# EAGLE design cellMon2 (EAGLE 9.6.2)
DATABASE: Z:\Eigene Dateien\Anwendungsdaten\Eagle\partdb\exp.txt

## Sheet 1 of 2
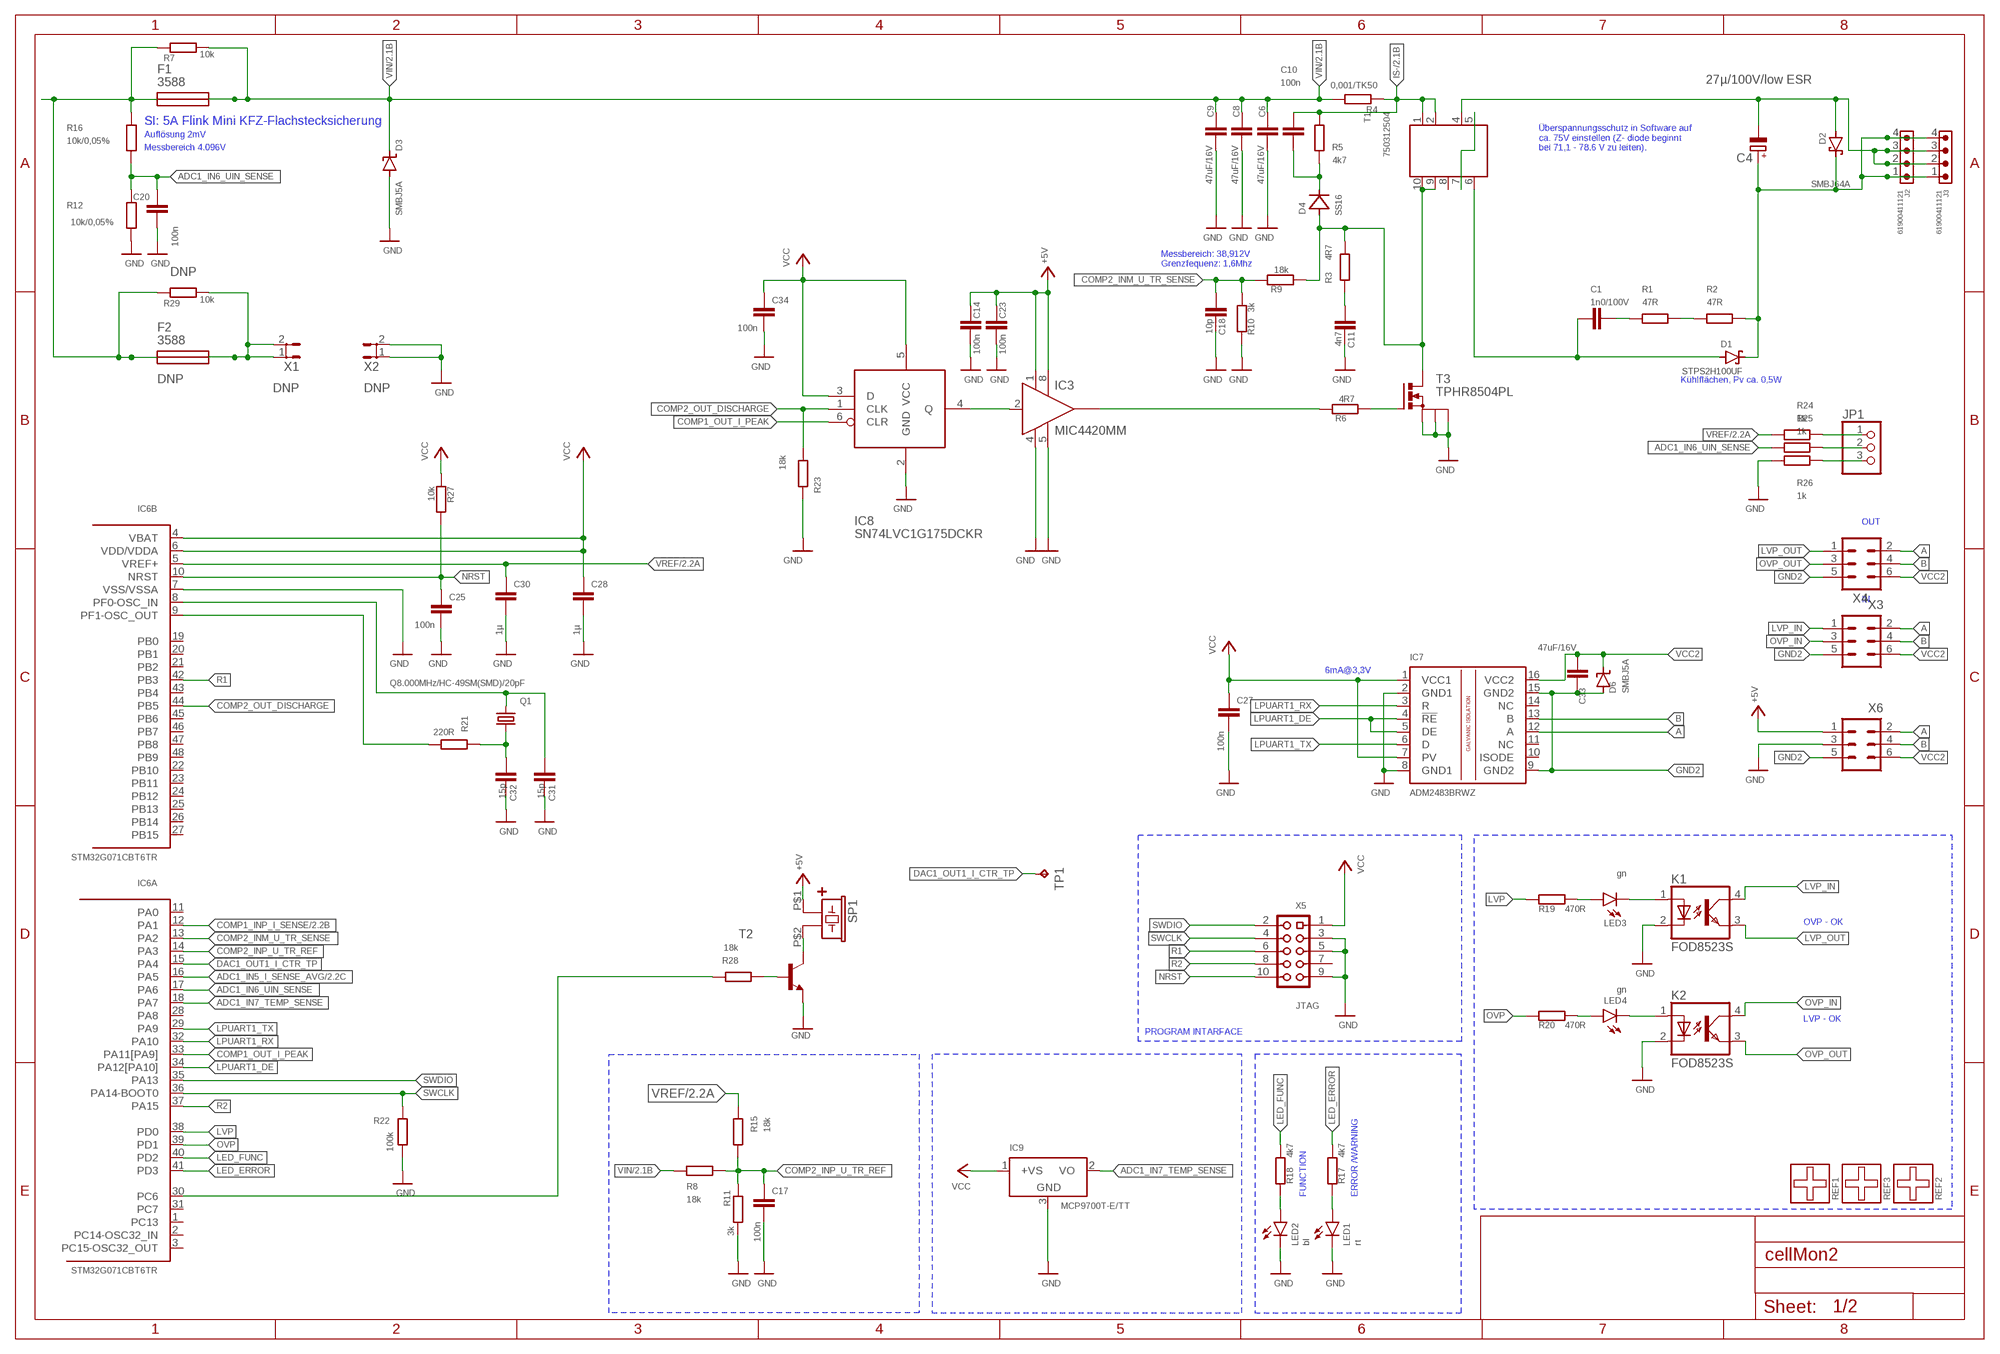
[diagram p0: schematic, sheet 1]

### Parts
C1  1n0/100V  C-EUC1206  [C1206]
C4  27µ/100V/low ESR  CPOL-EU153CLV-1010  [153CLV-1010]
C6  47uF/16V  C-EUC1210  [C1210]
C8  47uF/16V  C-EUC1210  [C1210]
C9  47uF/16V  C-EUC1210  [C1210]
C10  100n  C-EUC0603  [C0603]
C11  4n7  C-EUC0603K  [C0603K]
C14  100n  C-EUC0603K  [C0603K]
C17  100n  C-EUC0603K  [C0603K]
C18  10p  C-EUC0603  [C0603]
C20  100n  C-EUC0603K  [C0603K]
C23  100n  C-EUC0603K  [C0603K]
C25  100n  C-EUC0603K  [C0603K]
C27  100n  C-EUC0603K  [C0603K]
C28  1µ  C-EUC0603  [C0603]
C30  1µ  C-EUC0603  [C0603]
C31  15p  C-EUC0805  [C0805]
C32  15p  C-EUC0805  [C0805]
C33  47uF/16V  C-EUC1210  [C1210]
C34  100n  C-EUC0603K  [C0603K]
D1  STPS2H100UF  SCHOTTKY-DIODESMD  [SMB]
D2  SMBJ64A  SCHOTTKY-DIODESMD  [SMB]
D3  SMBJ5A  SUPPRESSOR-SMBJ  [SMBJ]
D4  SS16  MBRA340T3  [SMA]
D6  SMBJ5A  SUPPRESSOR-SMBJ  [SMBJ]
F1  3588  3588NORMAL  [3588]
F2  3588  3588NORMAL  [3588]
IC3  MIC4420MM  [MSOP8]
IC6  STM32G071CBT6TR  STM32G070CB  [LQFP48]
IC7  ADM2483BRWZ  ISO1176  [SO-16DW]
IC8  SN74LVC1G175DCKR  1G175  [SOT65P210X110-6N]
IC9  MCP9700T-E/TT  LM50  [SOT23]
J2  61900411121  61900411121  [61900411121]
J3  61900411121  61900411121  [61900411121]
JP1  PINHD-1X3  [1X03]
K1  FOD8523S  LTV816S  [SMD4]
K2  FOD8523S  LTV816S  [SMD4]
LED1  rt  LEDCHIPLED_0603  [CHIPLED_0603]
LED2  bl  LEDCHIPLED_0603  [CHIPLED_0603]
LED3  gn  LEDCHIPLED_0603  [CHIPLED_0603]
LED4  gn  LEDCHIPLED_0603  [CHIPLED_0603]
Q1  Q8.000MHz/HC-49SM(SMD)/20pF  CRYSTALHC49UP  [HC49UP]
R1  47R  R-EU_R1206  [R1206]
R2  47R  R-EU_R1206  [R1206]
R3  4R7  R-EU_R1206  [R1206]
R4  0,001/TK50  R-EU_R2512  [R2512]
R5  4k7  R-EU_R1206  [R1206]
R6  4R7  R-EU_R0603  [R0603]
R7  10k  R-EU_R0603  [R0603]
R8  18k  R-EU_R0603  [R0603]
R9  18k  R-EU_R0603  [R0603]
R10  3k  R-EU_R0603  [R0603]
R11  3k  R-EU_R0603  [R0603]
R12  10k/0,05%  R-EU_R0603  [R0603]
R15  18k  R-EU_R0603  [R0603]
R16  10k/0,05%  R-EU_R0603  [R0603]
R17  4k7  R-EU_R0603  [R0603]
R18  4k7  R-EU_R0603  [R0603]
R19  470R  R-EU_R0603  [R0603]
R20  470R  R-EU_R0603  [R0603]
R21  220R  R-EU_R0603  [R0603]
R22  100k  R-EU_R0603  [R0603]
R23  18k  R-EU_R0603  [R0603]
R24  1k  R-EU_R0603  [R0603]
R25  1k  R-EU_R0603  [R0603]
R26  1k  R-EU_R0603  [R0603]
R27  10k  R-EU_R0603  [R0603]
R28  18k  R-EU_R0603  [R0603]
R29  10k  R-EU_R0603  [R0603]
REF1  FIDUCIAL70UM_VERSION  [REF-DRUCK_FOR70UMCU]
REF2  FIDUCIAL70UM_VERSION  [REF-DRUCK_FOR70UMCU]
REF3  FIDUCIAL70UM_VERSION  [REF-DRUCK_FOR70UMCU]
SP1  LOUDITY_SPB45  [SPB45]
T1  750312504  WE-DSL_750050702  [WE_EP13_SMD_9PIN]
T2  MMBT2222ALT1-NPN-SOT23-BEC  [SOT23-BEC]
T3  TPHR8504PL  [DSOP8]
TP1  TPTP10R  [TP10R]
X1  ST6,3  [ST6,3]
X2  ST6,3  [ST6,3]
X3  ML6  [ML6]
X4  ML6  [ML6]
X5  JTAG  PF2X5SMD1.27MM  [PF2X5SMD50MIL]
X6  ML6  [ML6]

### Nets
+: C1.1 D1.A T1.6
+5V: C14.1 C23.1 IC3.1(VS) IC3.8(VS1) SP1.P$1(1P) X6.1 ; also sheet 2
+UB: F1.1A F1.1B F2.1A F2.1B R7.1 R16.1 R29.1
A: IC7.12(A) X3.2 X4.2 X6.2
ADC1_IN5_I_SENSE_AVG: IC6.16(A:PA5) ; also sheet 2
ADC1_IN6_UIN_SENSE: C20.1 IC6.17(A:PA6) R12.1 R16.2 R25.1
ADC1_IN6_UIN_SENSE_: JP1.2 R25.2
ADC1_IN7_TEMP_SENSE: IC6.18(A:PA7) IC9.2(VO)
B: IC7.13(B) X3.4 X4.4 X6.4
COMP1_INP_I_SENSE: IC6.12(A:PA1) ; also sheet 2
COMP1_OUT_I_PEAK: IC6.33(A:PA11[PA9]) IC8.6(CLR)
COMP2_INM_U_TR_SENSE: C18.1 IC6.13(A:PA2) R9.1 R10.2
COMP2_INP_U_TR_REF: C17.1 IC6.14(A:PA3) R8.2 R11.1 R15.2
COMP2_OUT_DISCHARGE: IC6.44(B:PB5) IC8.1(CLK) R23.2
DAC1_OUT1_I_CTR_TP: IC6.15(A:PA4) TP1.TP
GND: C6.2 C8.2 C9.2 C11.2 C14.2 C17.2 C18.2 C20.2 C23.2 C25.2 C27.2 C28.2 C30.2 C31.1 C32.1 C34.2 D3.A IC3.4(GND) IC3.5(GND1) IC6.7(B:VSS/VSSA) IC7.2(GND1) IC7.8(GND1) IC8.2(GND) IC9.3(GND) K1.2(C) K2.2(C) LED1.C LED2.C R10.1 R11.2 R12.2 R22.2 R23.1 R26.1 T2.E T3.S@1(S) T3.S@2(S) T3.S@3(S) X2.1 X2.2 X5.3 X5.5 X5.9 X6.3 ; also sheet 2
GND2: C33.1 D6.A IC7.9(GND2) IC7.15(GND2) X3.5 X4.5 X6.5
IS-: C10.1 R4.1 R5.2 T1.1 T1.2 ; also sheet 2
LED_ERROR: IC6.41(A:PD3) R17.1
LED_FUNC: IC6.40(A:PD2) R18.1
LPUART1_DE: IC6.34(A:PA12[PA10]) IC7.4(!RE) IC7.5(DE)
LPUART1_RX: IC6.32(A:PA10) IC7.3(R)
LPUART1_TX: IC6.29(A:PA9) IC7.6(D)
LVP: IC6.38(A:PD0) R19.1
LVP_IN: K1.4(COL) X3.1
LVP_OUT: K1.3(EMIT) X4.1
N$1: IC3.6(OUT) R6.1
N$2: R1.2 R2.1
N$3: C31.2 IC6.8(B:PF0-OSC_IN) Q1.2
N$5: C1.2 R1.1
N$7: C4.- D2.A J2.2 J2.3 J3.2 J3.3 T1.4
N$8: IC3.2(IN) IC8.4(Q)
N$9: IC6.9(B:PF1-OSC_OUT) R21.2
N$10: SP1.P$2(2N) T2.C
N$11: T1.5 T1.7
N$12: C32.2 Q1.1 R21.1
N$16: R28.2 T2.B
N$17: C4.+ D1.C D2.C J2.1 J2.4 J3.1 J3.4 R2.2
N$18: LED4.A R20.2
N$19: LED3.A R19.2
N$20: R6.2 T3.G
N$21: JP1.3 R26.2
N$23: C11.1 R3.1
N$24: D4.A R3.2 R9.2 T1.9 T1.10 T3.D
N$25: C10.2 D4.C R5.1
N$26: IC6.30(A:PC6) R28.1
N$28: F2.2A F2.2B R29.2 X1.1 X1.2
N$31: LED2.A R18.2
N$34: LED1.A R17.2
N$35: K2.1(A) LED4.C
N$36: K1.1(A) LED3.C
NRST: C25.1 IC6.10(B:NRST) R27.1 X5.10
OVP: IC6.39(A:PD1) R20.1
OVP_IN: K2.4(COL) X3.3
OVP_OUT: K2.3(EMIT) X4.3
R1: IC6.42(B:PB3) X5.6
R2: IC6.37(A:PA15) X5.8
SWCLK: IC6.36(A:PA14-BOOT0) R22.1 X5.4
SWDIO: IC6.35(A:PA13) X5.2
VCC: C27.1 C28.1 C34.1 IC6.4(B:VBAT) IC6.6(B:VDD/VDDA) IC7.1(VCC1) IC7.7(PV) IC8.3(D) IC8.5(VCC) IC9.1(+VS) R27.2 X5.1 ; also sheet 2
VCC2: C33.2 D6.C IC7.16(VCC2) X3.6 X4.6 X6.6
VIN: C6.1 C8.1 C9.1 D3.C F1.2A F1.2B R4.2 R7.2 R8.1 ; also sheet 2
VREF: C30.1 IC6.5(B:VREF+) R15.1 R24.1 ; also sheet 2
VREF_: JP1.1 R24.2
Unconnected: IC3.7(OUT) IC6.1(A:PC13) IC6.2(A:PC14-OSC32_IN) IC6.3(A:PC15-OSC32_OUT) IC6.11(A:PA0) IC6.19(B:PB0) IC6.20(B:PB1) IC6.21(B:PB2) IC6.22(B:PB10) IC6.23(B:PB11) IC6.24(B:PB12) IC6.25(B:PB13) IC6.26(B:PB14) IC6.27(B:PB15) IC6.28(A:PA8) IC6.31(A:PC7) IC6.43(B:PB4) IC6.45(B:PB6) IC6.46(B:PB7) IC6.47(B:PB8) IC6.48(B:PB9) IC7.10(ISODE) IC7.11(NC) IC7.14(NC) REF1.P$1 REF2.P$1 REF3.P$1 T1.8 X5.7

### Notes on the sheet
- SI: 5A Flink Mini KFZ-Flachstecksicherung
- Auflösung 2mV
- Messbereich 4.096V
- Überspannungsschutz in Software auf
  ca. 75V einstellen (Z- diode beginnt 
  bei 71,1 - 78.6 V zu leiten).
- Messbereich: 38,912V
- Grenzfequenz: 1,6Mhz
- Kühlflächen, Pv ca. 0,5W
- OUT
- IN
- 6mA@3,3V
- OVP - OK
- LVP - OK
- PROGRAM INTARFACE
- FUNCTION | ERROR /WARNING

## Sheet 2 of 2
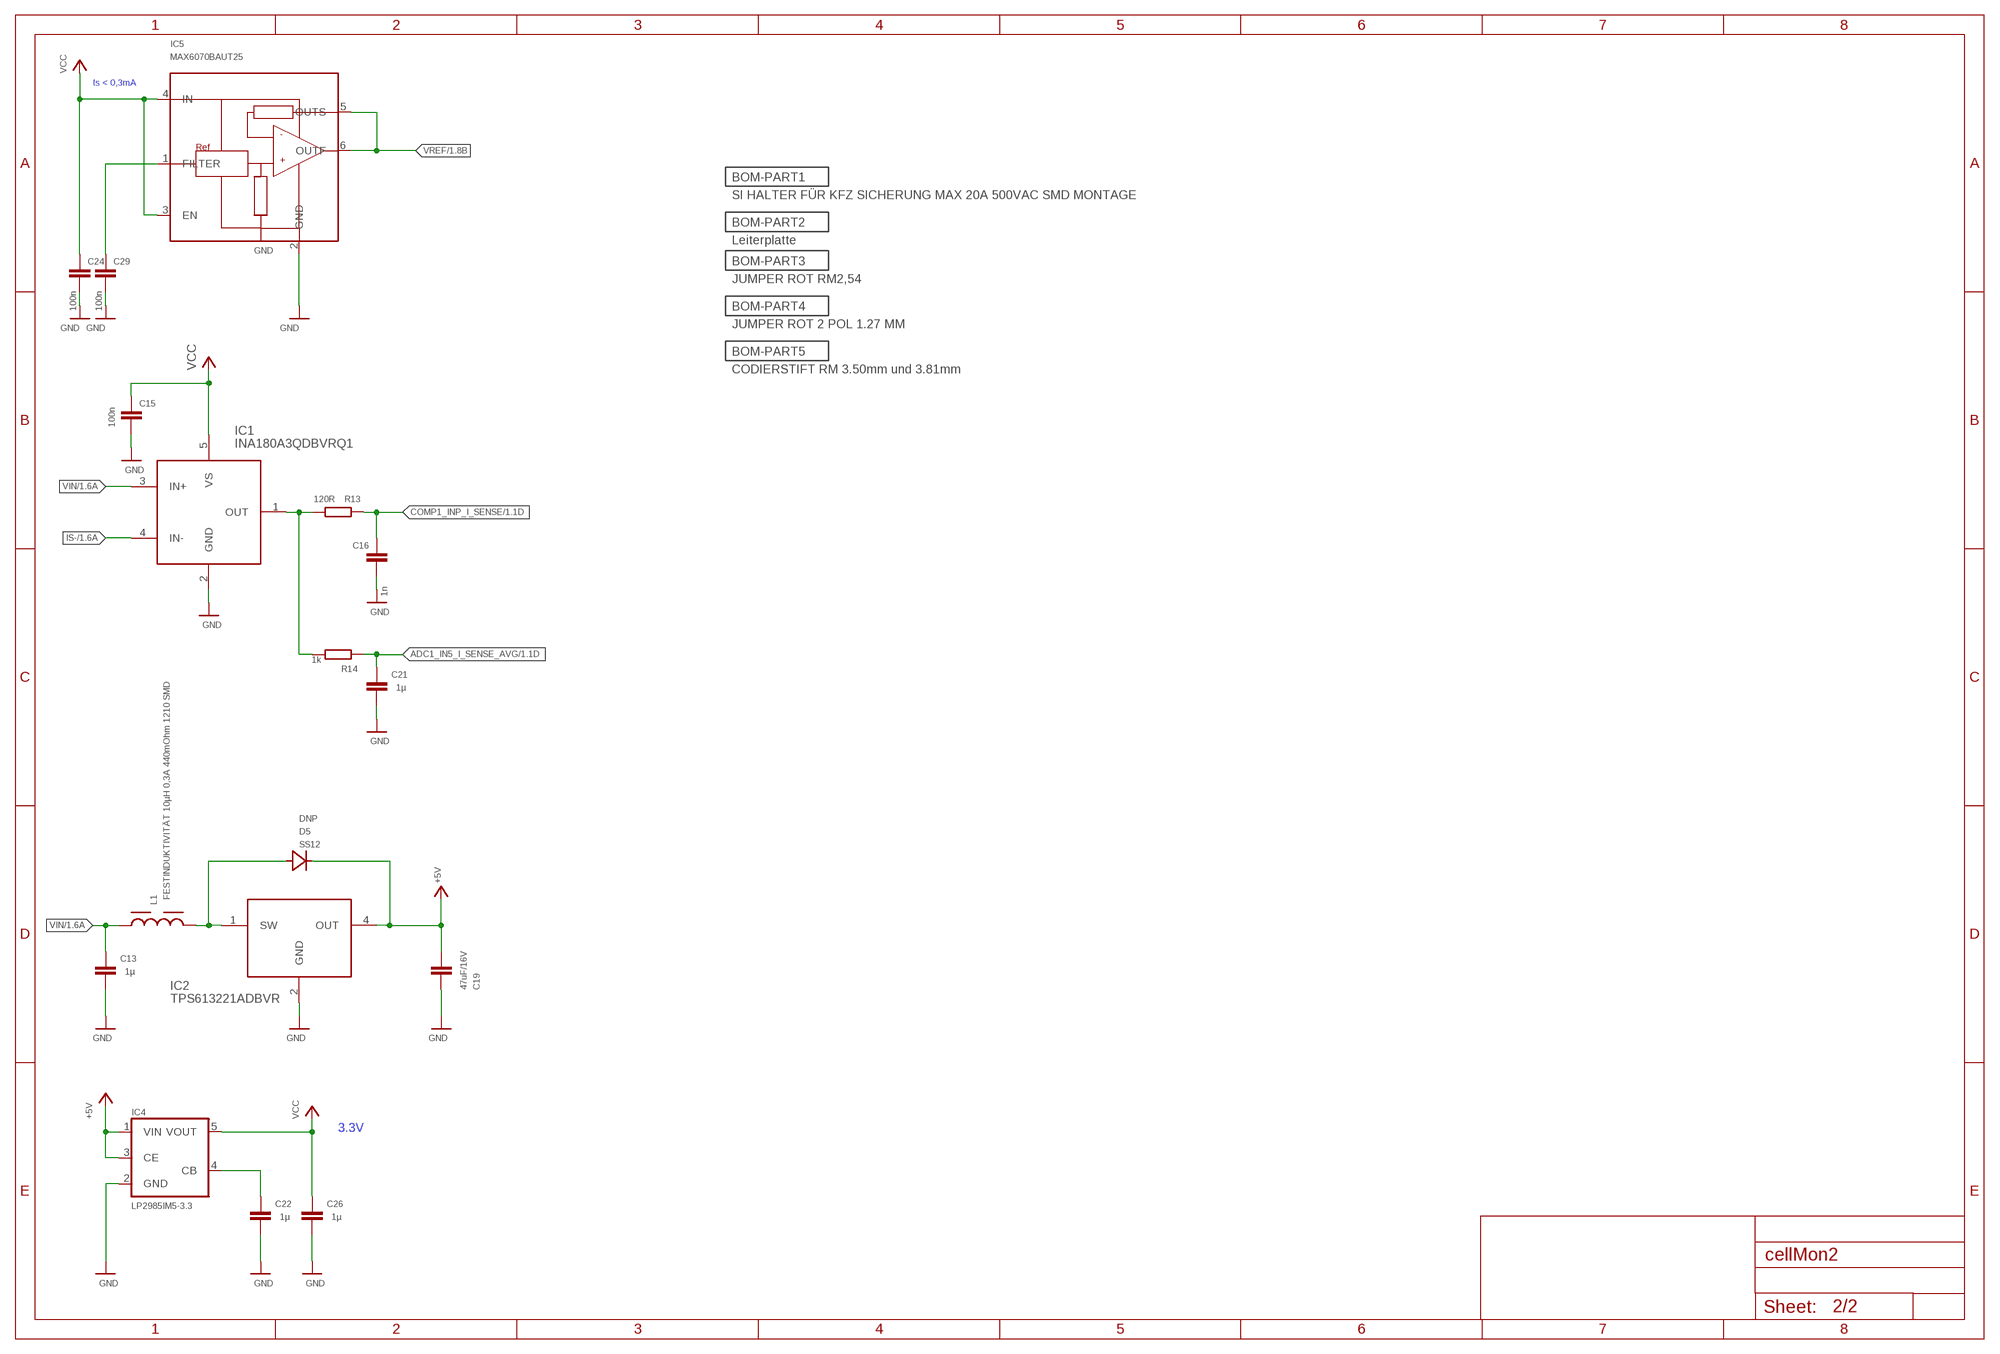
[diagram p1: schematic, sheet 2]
BOM-PART1 (BOM-PART): BOM: INCLUDE; PARTNO: EM008; QTY: 1
BOM-PART2 (BOM-PART): BOM: INCLUDE; PARTNO: PT057; QTY: 1
BOM-PART3 (BOM-PART): BOM: INCLUDE; PARTNO: CON085; QTY: 1
BOM-PART4 (BOM-PART): BOM: INCLUDE; PARTNO: CON363; QTY: 1
BOM-PART5 (BOM-PART): BOM: INCLUDE; PARTNO: CON441; QTY: 1

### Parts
C13  1µ  C-EUC0603  [C0603]
C15  100n  C-EUC0603K  [C0603K]
C16  1n  C-EUC0603  [C0603]
C19  47uF/16V  C-EUC1210  [C1210]
C21  1µ  C-EUC0603  [C0603]
C22  1µ  C-EUC0603  [C0603]
C24  100n  C-EUC0603K  [C0603K]
C26  1µ  C-EUC0603  [C0603]
C29  100n  C-EUC0603K  [C0603K]
D5  SS12  MBRA340T3  [SMA]
IC1  INA180A3QDBVRQ1  INA180A  [SOT95P280X110-5N]
IC2  TPS613221ADBVR  TPS613221ADBV  [SOT95P280X110-5N]
IC4  LP2985IM5-3.3  TS520529  [SOT25]
IC5  MAX6070BAUT25  MAX6070  [SOT23-6]
L1  FESTINDUKTIVITÄT 10µH 0,3A 440mOhm 1210 SMD  WE-LQS_3015_74404032022  [WE-LQS_3015]
R13  120R  R-EU_R0603  [R0603]
R14  1k  R-EU_R0603  [R0603]

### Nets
+5V: C19.1 D5.C IC2.4(OUT) IC4.1(VIN) IC4.3(CE) ; also sheet 1
ADC1_IN5_I_SENSE_AVG: C21.1 R14.1 ; also sheet 1
COMP1_INP_I_SENSE: C16.1 R13.1 ; also sheet 1
GND: C13.2 C15.2 C16.2 C19.2 C21.2 C22.2 C24.2 C26.2 C29.2 IC1.2(GND) IC2.2(GND) IC4.2(GND) IC5.2(GND) ; also sheet 1
IS-: IC1.4(IN-) ; also sheet 1
N$4: D5.A IC2.1(SW) L1.2
N$6: C22.1 IC4.4(CB)
N$14: IC1.1(OUT) R13.2 R14.2
N$22: C29.1 IC5.1(FILTER)
VCC: C15.1 C24.1 C26.1 IC1.5(VS) IC4.5(VOUT) IC5.3(EN) IC5.4(IN) ; also sheet 1
VIN: C13.1 IC1.3(IN+) L1.1 ; also sheet 1
VREF: IC5.5(OUTS) IC5.6(OUTF) ; also sheet 1

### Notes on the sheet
- Is < 0,3mA
- 3.3V

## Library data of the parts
C1 = rcl:C-EU: CAPACITOR, European symbol; PARTNO: C407; SPICEPREFIX: C
C4 = rcl:CPOL-EU: POLARIZED CAPACITOR, European symbol; PARTNO: C448; SPICEPREFIX: C
C6 C8 C9 C19 C33 = rcl:C-EU: CAPACITOR, European symbol; PARTNO: C219; SPICEPREFIX: C
C10 = rcl:C-EU: CAPACITOR, European symbol; PARTNO: C059; SPICEPREFIX: C
C11 = rcl:C-EU: CAPACITOR, European symbol; PARTNO: C051; SPICEPREFIX: C
C13 C21 C22 C26 C28 C30 = rcl:C-EU: CAPACITOR, European symbol; PARTNO: C079; SPICEPREFIX: C
C14 C15 C17 C20 C23-C25 C27 C29 C34 = rcl:C-EU: CAPACITOR, European symbol; PARTNO: C067; SPICEPREFIX: C
C16 = rcl:C-EU: CAPACITOR, European symbol; PARTNO: C043; SPICEPREFIX: C
C18 = rcl:C-EU: CAPACITOR, European symbol; PARTNO: C427; SPICEPREFIX: C
C31 C32 = resistor:C-EU: CAPACITOR, European symbol; PARTNO: C249
D1 = diode:SCHOTTKY-DIODE: Schottky Diode; PARTNO: D093
D2 = diode:SCHOTTKY-DIODE: Schottky Diode; PARTNO: D203
D3 D6 = diode:SUPPRESSOR-: Suppressor diode; PARTNO: D087
D4 = diode:MBRA340T3: Surface Mount Schottky Power Rectifier; PARTNO: D089
D5 = diode:MBRA340T3: Surface Mount Schottky Power Rectifier; DNP: T; PARTNO: D090
F1 = fuse_keystone_3568:3588; PARTNO: EM011
F2 = fuse_keystone_3568:3588; DNP: T; PARTNO: EM011
IC1 = ina180:INA180: Unidrectional current Sense Verstärkung 20/50/100/200; PARTNO: IC325
IC2 = TPS613221:TPS613221; PARTNO: IC328
IC3 = my_transistor-power:MIC4420: 6A-Peak Low-Side MOSFET Driver Bipolar/CMOS/DMOS Process http://www.micrel.com/_PDF/mic4420.pdf; PARTNO: IC039
IC4 = v-reg:TS5205: 150mA Low Noise LDO Voltage Regulator with Enable TSC [Taiwan Semiconductor Company, Ltd] Source: http://www.taiwansemi.com .. 5205_0409c.pdf; PARTNO: IC026
IC5 = max6070:MAX6070; PARTNO: IC326
IC6 = STM32G070CB:STM32G070CB: Arm® Cortex®-M0+ 32-bit MCU, 128 KB Flash, 36 KB RAM, 4x USART, timers, ADC, comm. I/Fs, 2.0-3.6V; PARTNO: IC321
IC7 = texas:ISO1176: ISOLATED RS-485 PROFIBUS TRANSCEIVER Source: Data sheet; MPN: ISO1176DW; OC_FARNELL: 1755037; OC_NEWARK: 13N4111; PARTNO: IC002
IC8 = 74LVC1G175:1G175: D Flip-Flop mit Reset im SC70 Gehäuse (6-pin); PARTNO: IC329
IC9 = linear:LM50: SOT-23 Single-Supply Centigrade Temperature Sensor Vout = (10mV/°C x Temp °C) +5mmmV Source: http://cache.national.com/ds/LM/LM50.pdf; PARTNO: IC040
J2 J3 = Wurth_Connectors_WR-WTB:61900411121: WR-WTB 2.54 mm Male Locking Header KIND PROPERTIES: Pitch:2.54 mm Gender:Male MATERIAL PROPERTIES: Insulator Material :PA66 Insulator Flammability Rating:UL94 V-0 Insulator Color:Beige Contact Material:Copper Alloy Contact Plating:Tin Contact Type:Stamped GENERAL INFORMATION Operating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; CONTACT-RESISTANCE: 20mOhm; DATASHEET-URL: https://www.we-online.com/redexpert/spec/61900411121?ae; GENDER: Male; L: 10.16mm; MOUNT: THT; PACKAGING: Bag; PART-NUMBER: 61900411121; PCB-CABLE-PANEL: PCB; PINS: 4; PITCH: 2.54mm; TYPE: Vertical; WORKING-VOLTAGE: 250V(AC)
JP1 = pinhead:PINHD-1X3: PIN HEADER; PARTNO: CON031
K1 K2 = optocoupler:LTV816: OPTO COUPLER Source: LITEON, LTV816.pdf; OC_FARNELL: unknown; OC_NEWARK: unknown; PARTNO: IC053
L1 = Wurth_Power Magnetics_WE-LQS:WE-LQS_3015: WE-LQS SMD Power Inductor; DATASHEET-URL: https://www.we-online.com/catalog/datasheet/74404032022.pdf; FRES: 75MHz; IR: 1.8A; ISAT: 1.7A; PART-NUMBER: 74404032022; PARTNO: L114; RDC: 50mOhm; VALUE: uH2.2
LED1 = led:LED: LED; PARTNO: D079
LED2 = led:LED: LED; PARTNO: D077
LED3 LED4 = led:LED: LED; PARTNO: D078
Q1 = crystal:CRYSTAL: CRYSTAL; OC_FARNELL: unknown; OC_NEWARK: unknown; PARTNO: Q003
R1 R2 = rcl:R-EU_: RESISTOR, European symbol; PARTNO: R574; SPICEPREFIX: R
R3 = rcl:R-EU_: RESISTOR, European symbol; PARTNO: R550; SPICEPREFIX: R
R4 = rcl:R-EU_: RESISTOR, European symbol; PARTNO: R826; SPICEPREFIX: R
R5 = rcl:R-EU_: RESISTOR, European symbol; PARTNO: R622; SPICEPREFIX: R
R6 = rcl:R-EU_: RESISTOR, European symbol; PARTNO: R141; SPICEPREFIX: R
R7 R27 = rcl:R-EU_: RESISTOR, European symbol; PARTNO: R221; SPICEPREFIX: R
R8 R9 R15 R23 R28 = rcl:R-EU_: RESISTOR, European symbol; PARTNO: R227; SPICEPREFIX: R
R10 R11 = rcl:R-EU_: RESISTOR, European symbol; PARTNO: R208; SPICEPREFIX: R
R12 R16 = rcl:R-EU_: RESISTOR, European symbol; PARTNO: R869; SPICEPREFIX: R
R13 = rcl:R-EU_: RESISTOR, European symbol; PARTNO: R175; SPICEPREFIX: R
R14 R24-R26 = rcl:R-EU_: RESISTOR, European symbol; PARTNO: R197; SPICEPREFIX: R
R17 R18 = rcl:R-EU_: RESISTOR, European symbol; PARTNO: R213; SPICEPREFIX: R
R19 R20 = rcl:R-EU_: RESISTOR, European symbol; PARTNO: R189; SPICEPREFIX: R
R21 = resistor:R-EU_: RESISTOR, European symbol; PARTNO: R181
R22 = resistor:R-EU_: RESISTOR, European symbol; PARTNO: R245
R29 = rcl:R-EU_: RESISTOR, European symbol; DNP: T; PARTNO: R221; SPICEPREFIX: R
REF1-REF3 = Fiducial (1):FIDUCIAL; BOM: EXCLUDE
SP1 = mBuzzer:LOUDITY_SPB45
T1 = Wuerth_Elektronik_eiSos_V6:WE-DSL_750050702: SMD-ADSL Transformer WE-DSL - IEC60950 compatible -- for ADSL applications -- Matched to various manufacturers ADSL ICs; PARTNO: L096
T2 = transistor:*-NPN-: NPN Transistror BF959 corrected 2008.03.06
T3 = TPW_MOSFET:TPHR8504PL; PARTNO: T134
TP1 = testpad:TP: Test pad
X1 X2 = con-rib:ST6,3: RIBBON CABLE CONNECTOR; DNP: T; OC_FARNELL: unknown; OC_NEWARK: unknown
X3 X4 X6 = con-harting-ml:ML6: HARTING; OC_FARNELL: unknown; OC_NEWARK: unknown; PARTNO: CON207
X5 = A_CONN:PF2X5; PARTNO: CON156

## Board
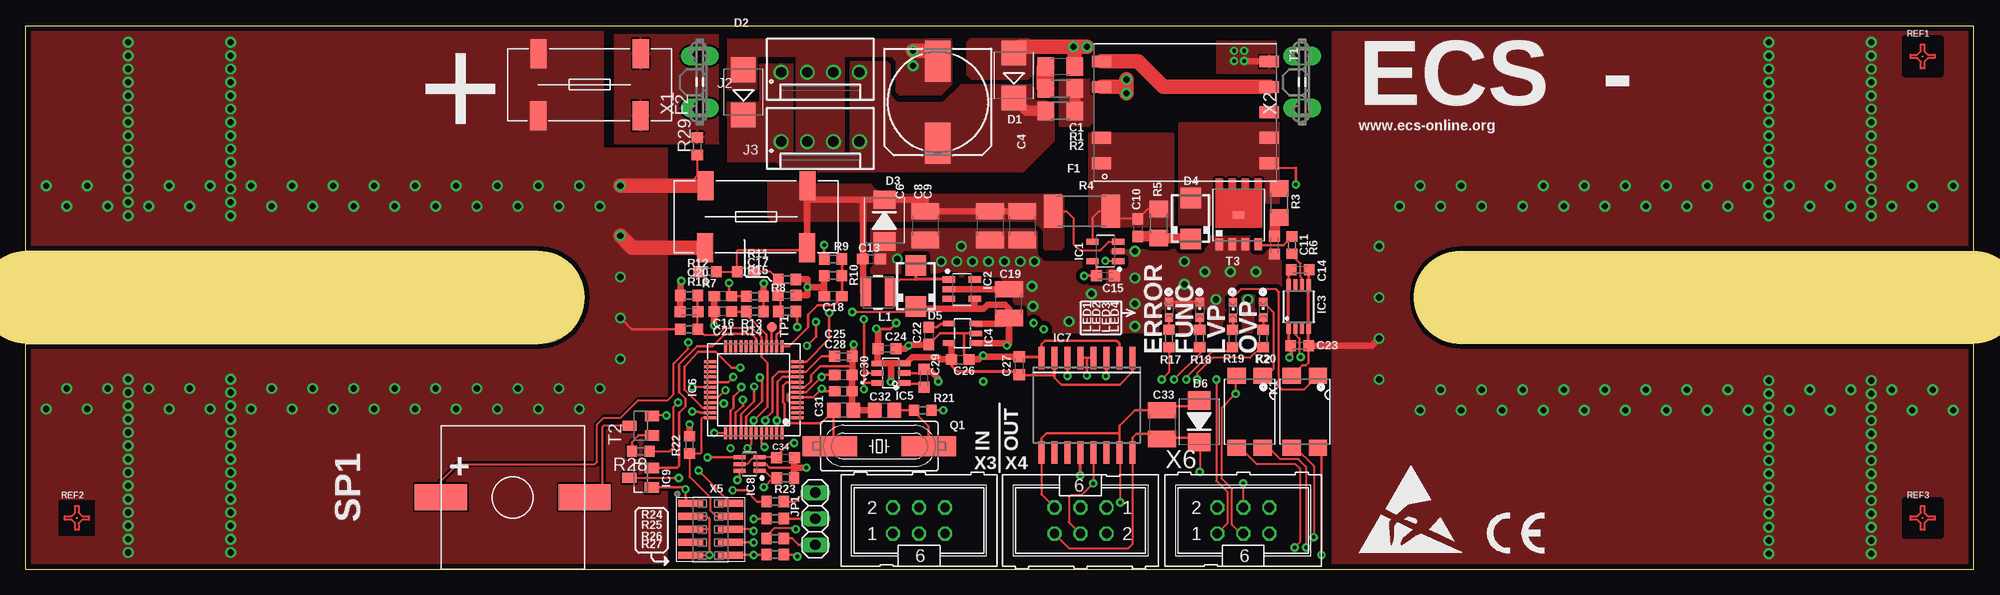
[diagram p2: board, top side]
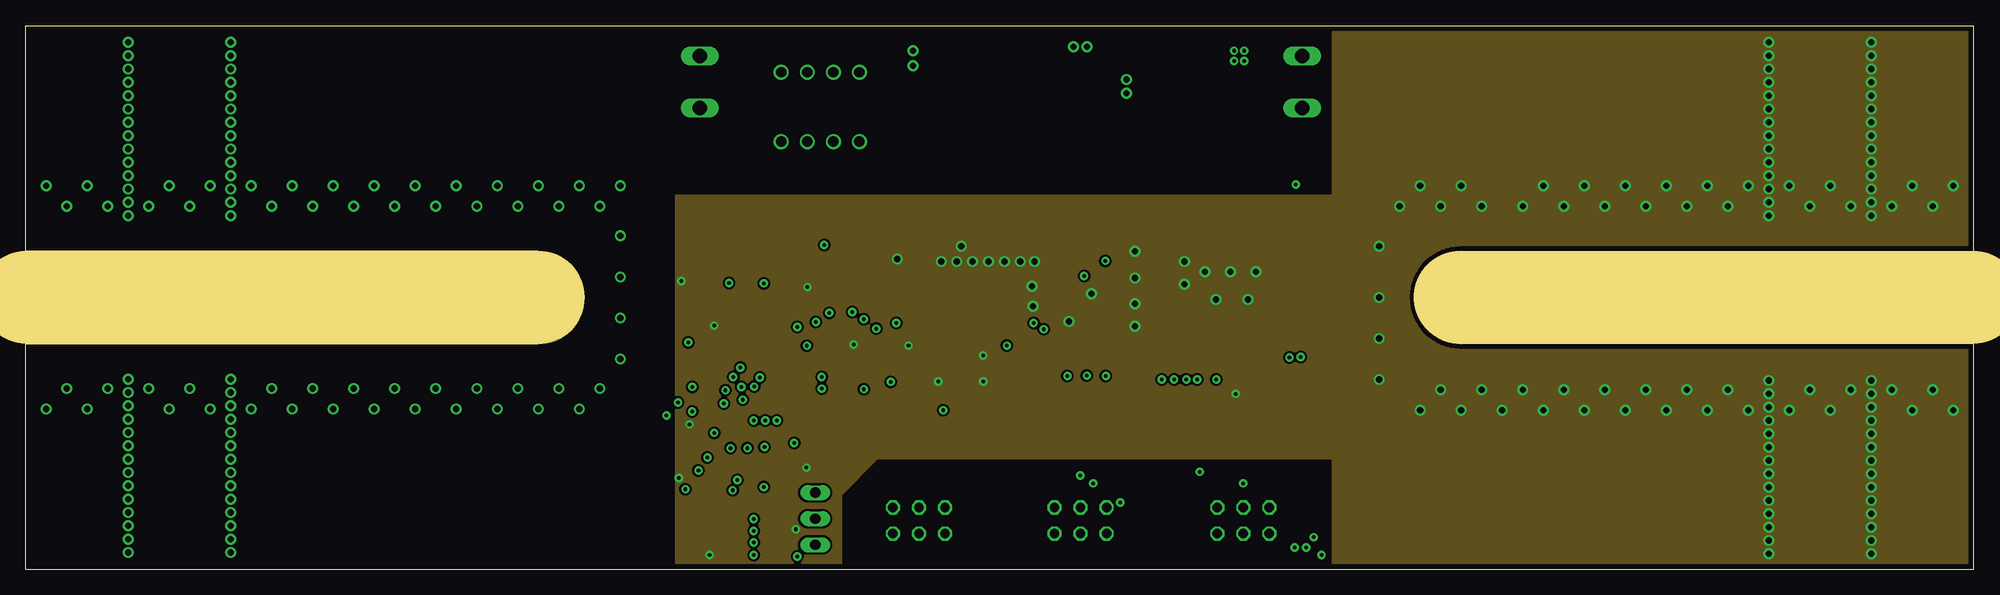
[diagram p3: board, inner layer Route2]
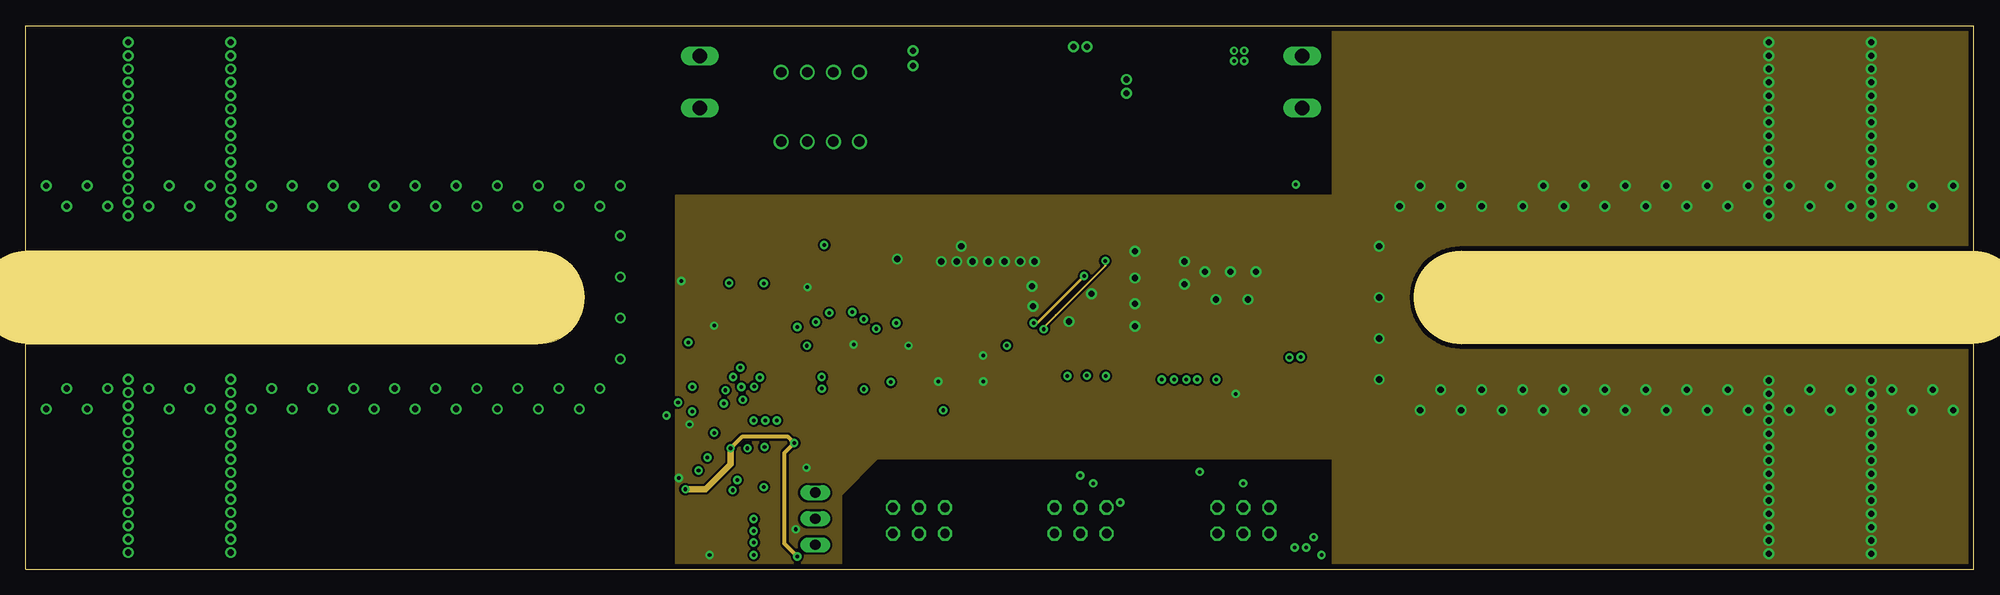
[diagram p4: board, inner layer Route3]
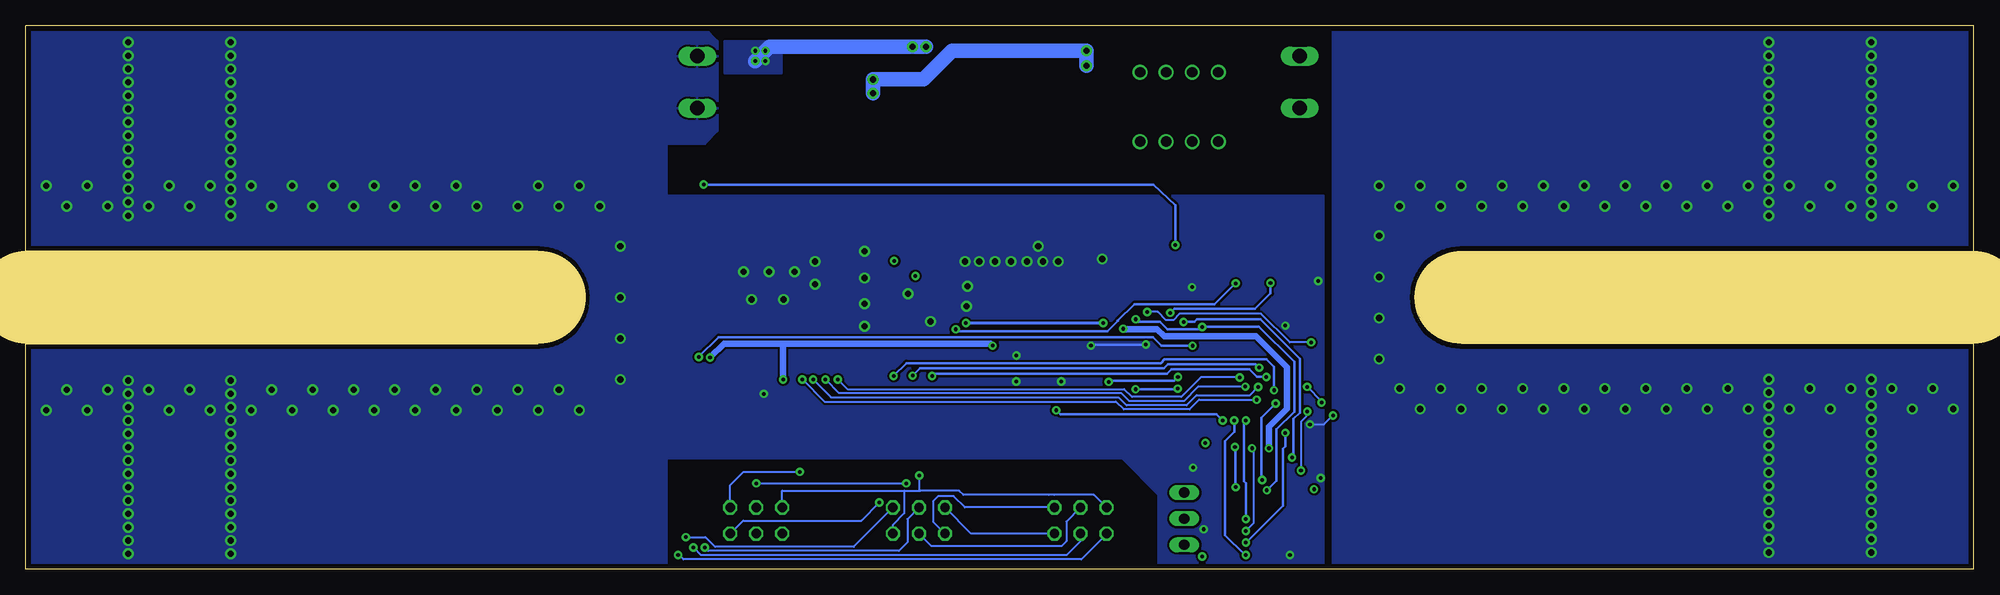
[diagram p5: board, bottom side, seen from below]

Size 190 x 53 mm. Coordinates in mm from the lower left corner, seen from the top.
Outline: 0,0 190,0 190,22 140,22 arc-180 140,31 190,31 190,53 0,53 0,31 50,31 arc-180 50,22 0,22 0,0
Copper layers (1+2*3+16): Top 0.018mm / dielectric 0.36mm / Route2 0.035mm / dielectric 0.71mm / Route3 0.035mm / dielectric 0.36mm / Bottom 0.018mm
Design rules "multi-cb_070um-cu *": minimum track width 8mil, minimum drill 12mil, track to track 8mil, track to pad 8mil, pad to pad 8mil, via to via 8mil, smd to smd 8mil, copper to edge 20mil, drill to drill 8mil, minimum pad ring 9mil, minimum via ring 9mil, stop-mask expansion 3mil, vias tented up to drill 0mil, thermal gap 8mil
Milling: 2 lines

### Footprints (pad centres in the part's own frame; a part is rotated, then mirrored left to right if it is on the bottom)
C1206 = smd 1.6 x 1.8: 1 -1.4,0; 2 1.4,0
153CLV-1010 = smd 4 x 2.5: + 4,0; - -4,0
C1210 = smd 1.6 x 2.7: 1 -1.4,0; 2 1.4,0
C0603 = smd 1.1 x 1: 1 -0.85,0; 2 0.85,0
C0603K = smd 1.05 x 1.08: 1 -0.875,0; 2 0.875,0
C0805 = smd 1.3 x 1.5: 1 -0.95,0; 2 0.95,0
SMB = smd 2.4 x 2.4: A 2.2,0; C -2.2,0
SMBJ = smd 1.78 x 2.16: A 2.04,0; C -2.03,0
SMA = smd 2 x 2: A 2,0; C -2,0
3588 = smd 1.57 x 2.82: 1A -4.955,3.03; 1B -4.995,-3.03; 2A 4.995,3.03; 2B 4.955,-3.03
SOT95P280X110-5N = smd 1.209 x 0.589: 1 -1.253,0.95; 2 -1.253,0; 3 -1.253,-0.95; 4 1.253,-0.95; 5 1.253,0.95
MSOP8 = smd 0.4 x 1.2: 1 -0.975,-2.05; 2 -0.325,-2.05; 3 0.325,-2.05; 4 0.975,-2.05; 5 0.975,2.05; 6 0.325,2.05; 7 -0.325,2.05; 8 -0.975,2.05
SOT25 = smd 0.55 x 1.2: 1 -0.95,-1.3; 2 0,-1.3; 3 0.95,-1.3; 4 0.95,1.3; 5 -0.95,1.3
SOT23-6 = smd 0.55 x 1.2: 1 -0.95,-1.3; 2 0,-1.3; 3 0.95,-1.3; 4 0.95,1.3; 5 0,1.3; 6 -0.95,1.3
LQFP48 = smd 0.29 x 1.2: 1 -2.75,-4.25; 2 -2.25,-4.25; 3 -1.75,-4.25; 4 -1.25,-4.25; 5 -0.75,-4.25; 6 -0.25,-4.25; 7 0.25,-4.25; 8 0.75,-4.25; 9 1.25,-4.25; 10 1.75,-4.25; 11 2.25,-4.25; 12 2.75,-4.25; 25 2.75,4.25; 26 2.25,4.25; 27 1.75,4.25; 28 1.25,4.25; 29 0.75,4.25; 30 0.25,4.25; 31 -0.25,4.25; 32 -0.75,4.25; 33 -1.25,4.25; 34 -1.75,4.25; 35 -2.25,4.25; 36 -2.75,4.25 | smd 1.2 x 0.29: 13 4.25,-2.75; 14 4.25,-2.25; 15 4.25,-1.75; 16 4.25,-1.25; 17 4.25,-0.75; 18 4.25,-0.25; 19 4.25,0.25; 20 4.25,0.75; 21 4.25,1.25; 22 4.25,1.75; 23 4.25,2.25; 24 4.25,2.75; 37 -4.25,2.75; 38 -4.25,2.25; 39 -4.25,1.75; 40 -4.25,1.25; 41 -4.25,0.75; 42 -4.25,0.25; 43 -4.25,-0.25; 44 -4.25,-0.75; 45 -4.25,-1.25; 46 -4.25,-1.75; 47 -4.25,-2.25; 48 -4.25,-2.75
SO-16DW = smd 0.6 x 2.2: 1 -4.445,-4.6; 2 -3.175,-4.6; 3 -1.905,-4.6; 4 -0.635,-4.6; 5 0.635,-4.6; 6 1.905,-4.6; 7 3.175,-4.6; 8 4.445,-4.6; 9 4.445,4.6; 10 3.175,4.6; 11 1.905,4.6; 12 0.635,4.6; 13 -0.635,4.6; 14 -1.905,4.6; 15 -3.175,4.6; 16 -4.445,4.6
SOT65P210X110-6N = smd 1.186 x 0.397: 1 -0.962,0.65; 2 -0.962,0; 3 -0.962,-0.65; 4 0.962,-0.65; 5 0.962,0; 6 0.962,0.65
SOT23 = smd 1 x 1.4: 1 -0.95,-1.1; 2 0.95,-1.1; 3 0,1.1
61900411121 = drill 1: 1 3.81,0.3; 2 1.27,0.3; 3 -1.27,0.3; 4 -3.81,0.3
1X03 = drill 1.016 long: 1 -2.54,0; 2 0,0; 3 2.54,0
SMD4 = smd 1.78 x 1.55: 1 -1.27,-3.5; 2 1.27,-3.5; 3 1.27,3.5; 4 -1.27,3.5
WE-LQS_3015 = smd 1 x 2.7: 1 -1.2,0; 2 1.2,0
CHIPLED_0603 = smd 0.8 x 0.8: A 0,-0.75; C 0,0.75
HC49UP = smd 5.334 x 1.93: 1 -4.826,0; 2 4.826,0
R1206 = smd 1.6 x 1.803: 1 -1.422,0; 2 1.422,0
R2512 = smd 1.8 x 3.2: 1 -2.8,0; 2 2.8,0
R0603 = smd 1 x 1.1: 1 -0.85,0; 2 0.85,0
REF-DRUCK_FOR70UMCU = smd 0.21 x 0.21: P$1 0,0
SPB45 = smd 2.54 x 5.08: P$1 0,7; P$2 0,-7
WE_EP13_SMD_9PIN = smd 1.88 x 1.143: 1 -8.18,-4.96; 2 -8.18,-2.48; 4 -8.18,2.48; 5 -8.18,4.96; 6 8.18,4.96; 7 8.18,2.48; 8 8.18,0; 9 8.18,-2.48; 10 8.18,-4.96
SOT23-BEC = smd 1 x 1.4: B -0.95,-1.1; C 0,1.1; E 0.95,-1.1
DSOP8 = smd 1.15 x 0.75: D 0,0 | smd 0.75 x 1.15: G 1.905,-2.875; S@1 -1.905,-2.875; S@2 -0.635,-2.875; S@3 0.635,-2.875
TP10R = smd 1 x 1: TP 0,0
ST6,3 = drill 1.397 long: 1 -2.54,0; 2 2.54,0
ML6 = drill 0.914 octagon: 1 -2.54,-1.27; 2 -2.54,1.27; 3 0,-1.27; 4 0,1.27; 5 2.54,-1.27; 6 2.54,1.27
PF2X5SMD50MIL = smd 0.7 x 2.4: 1 -2.54,-1.95; 2 -2.54,1.95; 3 -1.27,-1.95; 4 -1.27,1.95; 5 0,-1.95; 6 0,1.95; 7 1.27,-1.95; 8 1.27,1.95; 9 2.54,-1.95; 10 2.54,1.95

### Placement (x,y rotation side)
C1  100.9,49 180 top
C4  88.95,45.55 270 top
C6  87.75,33.5 270 top
C8  94.05,33.5 270 top
C9  97.2,33.5 270 top
C10  108.45,33.3 270 top
C11  121.8,31.6 270 top
C13  82.5,30.25 0 top
C14  124.3,29.2 0 top
C15  105.3,28.6 0 top
C16  68,26.62 180 top
C17  74.25,26.7 0 top
C18  78.75,26.62 180 top
C19  95.9,25.9 90 top
C20  64.7,25.1 180 top
C21  68,25.12 180 top
C22  88.08,22.75 270 top
C23  124.25,21.8 0 top
C24  84,21.5 0 top
C25  79.75,20.75 0 top
C26  91.15,20.45 0 top
C27  96.9,19.85 90 top
C28  79.75,18.95 0 top
C29  87.6,18.62 90 top
C30  79.75,17.35 0 top
C31  79.75,15.5 180 top
C32  83.75,15.5 0 top
C33  110.83,14.1 270 top
C34  74.1,10.85 0 top
D1  96.38,48.15 90 top
D2  70,46.5 90 top
D3  83.75,34 270 top
D4  113.6,34.2 90 top
D5  86.8,27.6 90 top
D6  114.45,14.4 90 top
F1  71.25,34.38 0 top
F2  55,47.25 0 top
IC1  105.3,31 180 top
IC2  91.3,27.3 0 top
IC3  124.15,25.6 0 top
IC4  91.35,23 90 top
IC5  84.38,19.12 90 top
IC6  71,17.5 90 top
IC7  103.5,16 180 top
IC8  70.6,10.25 180 top
IC9  59.98,8.93 90 top
J2  77.5,48.75 180 top
J3  77.5,42 180 top
JP1  77,4.93 270 top
K1  124.75,15.35 180 top
K2  119.38,15.35 180 top
L1  83.12,27 0 top
LED1  111.5,25.3 0 top
LED2  114.5,25.3 0 top
LED3  117.75,25.25 0 top
LED4  120.7,25.3 0 top
Q1  83.25,12 180 top
R1  100.9,46.85 0 top
R2  100.9,44.7 180 top
R3  122.25,35.7 90 top
R4  103,34.9 180 top
R5  110.5,33.7 90 top
R6  123.5,31.6 90 top
R7  66.5,29 0 top
R8  70.25,29 0 top
R9  78.75,30.25 180 top
R10  78.75,28.62 0 top
R11  74.25,28.25 0 top
R12  64.7,26.7 180 top
R13  71.12,26.62 0 top
R14  71.12,25.12 0 top
R15  74.25,25.12 180 top
R16  64.7,23.4 0 top
R17  111.5,22.5 90 top
R18  114.5,22.5 90 top
R19  117.7,22.5 90 top
R20  120.7,22.5 90 top
R21  87.5,15.5 0 top
R22  64.75,12.12 90 top
R23  74.1,8.9 180 top
R24  73.1,6.6 0 top
R25  73.1,4.95 0 top
R26  73.1,3 0 top
R27  73.1,1.43 0 top
R28  60,11.5 180 top
R29  65.5,41.25 90 top
REF1  185,50 0 top
REF2  5,5 0 top
REF3  185,5 0 top
SP1  47.5,7 90 top
T1  113.1,44.55 0 top
T2  60,14 90 top
T3  118.3,34.55 0 top
TP1  72.75,23.62 0 top
U$1  [ESD_10.00]  130,1.5 0 top
U$2  [CE-4MM]  142.5,1.5 0 top
X1  65.75,47.5 90 top
X2  124.5,47.5 90 top
X3  87.12,4.75 0 top
X4  102.88,4.75 180 top
X5  66.8,3.9 270 top
X6  118.75,4.75 0 top

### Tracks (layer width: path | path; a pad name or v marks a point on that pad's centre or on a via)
+  (via drill 0.35, 0.6)
  Top 0.61: T1.6 118.89,49.51 v118.85,49.55
  Top 1.422: C1.1 102.3,50.85 v102.2,50.95 | D1.A 96.97,50.95 v102.2,50.95 | v102.2,50.95 v103.5,50.95
  Bottom 1.422: v118.85,49.55 117.45,50.95 v102.2,50.95
  other vias: 118.85,50.55 117.85,50.55 117.85,49.55
  pour Top (no thermals): 92.2,51.7 97.85,51.7 98.3,51.25 98.3,48.35 97.7,47.75 92.3,47.75 91.85,48.2 91.85,51.35
  pour Top: 116.25,51.5 121.88,51.5 121.88,48.38 116.25,48.38
  pour Bottom: 116.25,51.5 121.88,51.5 121.88,48.38 116.25,48.38
+5V  (via drill 0.35)
  Top 0.203: X6.1 117.25,4.52 117.25,7.5 116.12,8.62 v116.12,18.5 | SP1.P$1 40.5,8.62 42.12,10.25 55.5,10.25 55.75,10.5 55.75,14.12 56.38,14.75 58,14.75 59.75,16.5 62.62,16.5 63.19,17.06 63.19,20.05 64.62,21.49 v64.62,22.12 | v80.62,25.08 86.28,25.08 D5.C
  Top 0.305: C23.1 123.17,22 IC3.1 IC3.8 123.17,28.95 C14.1
  Top 0.406: C23.1 123.38,20.77 v123.25,20.65
  Top 0.61: D5.C 87,25.4 92.6,25.4 | C19.1 95.9,25.4 95.5,25.8 93.8,25.8 93.4,25.4 92.6,25.4 | IC4.3 95.35,23.95 C19.1 | IC4.1 95.45,22.05 v95.7,21.8 95.9,22 C19.1 | IC2.4 92.55,25.45 92.6,25.4
  Bottom 0.203: v64.62,22.12 66.71,22.12 69.5,24.92 77.46,24.92 78.08,24.29 78.79,24.29 79.58,25.08 v80.62,25.08
  Bottom 0.61: v123.25,20.65 121.9,22 116.12,22 | 116.12,22 v116.12,18.5 | v95.7,21.8 95.9,22 116.12,22
+UB  (via drill 0.6)
  Top 0.203: R29.1 65.5,38.36 64.52,37.38
  Top 0.254: F1.1B 65.65,30.74 R7.1 | R16.1 59.1,23.4 v58,24.5
  Top 1.422: v58,37.38 64.52,37.38 66.27,37.38 F1.1A | v58,32.5 59.16,31.34 F1.1B
  other vias: 28,35.38 30,37.38 32,35.38 34,37.38 36,35.38 40,35.38 42,37.38 44,35.38 46,37.38 22,37.38 26,37.38 24,35.38 38,37.38 48,35.38 50,37.38 20,51.38 20,50.08 20,48.77 20,47.48 20,46.17 20,44.88 20,43.58 20,42.27 20,40.98 20,39.67 20,38.38 20,37.08 20,35.77 20,34.48 8,35.38 12,35.38 14,37.38 16,35.38 2,37.38 6,37.38 4,35.38 18,37.38 20,18.52 20,17.23 20,15.93 20,14.62 20,13.32 20,12.03 20,10.72 20,9.43 20,8.12 20,6.82 20,5.52 20,4.23 20,2.93 20,1.62 12,17.62 8,17.62 6,15.62 4,17.62 18,15.62 14,15.62 16,17.62 2,15.62 44,17.62 42,15.62 40,17.62 38,15.62 36,17.62 32,17.62 30,15.62 28,17.62 26,15.62 50,15.62 46,15.62 48,17.62 34,15.62 24,17.62 22,15.62 52,17.62 54,15.62 56,17.62 58,20.5 52,35.38 56,35.38 54,37.38 58,28.5 10,51.38 10,50.08 10,48.77 10,47.48 10,46.17 10,44.88 10,43.58 10,42.27 10,40.98 10,39.67 10,38.38 10,37.08 10,35.77 10,34.48 10,18.52 10,17.23 10,15.93 10,14.62 10,13.32 10,12.03 10,10.72 10,9.43 10,8.12 10,6.82 10,5.52 10,4.23 10,2.93 10,1.62
  pour Top (no thermals): 62.5,0 62.5,41 56.25,41 56.25,53 0,53 0,0
  pour Bottom (no thermals): 62.5,53 0,53 0,0 62.5,0
A  (via drill 0.35)
  Top 0.305: v102.85,9.15 102.85,11.38 IC7.12
  Bottom 0.203: X3.2 85.83,7.26 89.7,7.26 90.21,7.25 98.55,7.25 98.96,7.66 102.75,7.66 | 104.31,7.66 104.31,5.44 105.41,4.34 X4.2 | v102.85,9.15 102.85,7.76 102.75,7.66 | X6.2 116.21,7.66 104.31,7.66 | 104.31,7.66 102.75,7.66
ADC1_IN5_I_SENSE_AVG
  Top 0.254: IC6.16 72.25,22.86 70.25,24.86 R14.1 C21.1
ADC1_IN6_UIN_SENSE  (via drill 0.35)
  Top 0.203: 70.86,23.52 68.16,23.52 67.44,22.8 66.19,22.8 65.58,23.43 | R16.2 65.55,25.07 C20.1
  Top 0.254: v71,14.5 72.35,15.85 72.35,20.1 71.75,20.7 IC6.17 71.75,22.63 70.86,23.52 | R25.1 72.2,4.9 v71,4.9 | R12.1 65.55,25.12 C20.1 | 65.58,23.43 R16.2
  Bottom 0.254: v71,14.5 71.2,14.3 71.2,8.6 71,8.4 v71,4.9
ADC1_IN6_UIN_SENSE_
  Top 0.254: JP1.2 73.97,4.93 R25.2
ADC1_IN7_TEMP_SENSE
  Top 0.254: IC6.18 71.25,22.48 70.78,22.95 68.2,22.95 67,21.75 65.5,21.75 63.74,19.99 63.75,17.25 64.38,16.62 64.38,15.88 63.75,15.25 63.75,10.07 63.55,9.88 IC9.2
B  (via drill 0.35)
  Top 0.203: IC7.13 v104.12,8.38 103,7.25 102,7.25 101.75,7 101.75,4.61 X4.4 | X6.4 v118.75,8.38
  Bottom 0.203: X3.4 88.5,4.64 88.5,2.75 89,2.25 101.64,2.25 X4.4 | v118.75,8.38 v104.12,8.38
COMP1_INP_I_SENSE  (via drill 0.35)
  Top 0.254: IC6.12 76.17,20.25 78.38,22.45 v78.38,25 | R13.1 C16.1 68.6,26.7 v68.6,27.9
  Bottom 0.254: v78.38,25 77.97,25.4 70.1,25.4 68.6,26.9 v68.6,27.9
COMP1_OUT_I_PEAK  (via drill 0.35)
  Top 0.254: v69.4,8.71 69.64,8.95 IC8.6 | v68.1,16.15 68,16.25 IC6.33
  Bottom 0.254: v68.1,16.15 69.5,14.75 69.5,8.81 v69.4,8.71
COMP2_INM_U_TR_SENSE
  Top 0.254: IC6.13 74.45,21.75 76.3,23.6 76.3,24.8 77.25,25.75 78.85,25.75 79,25.9 C18.1 R10.2 R9.1
COMP2_INP_U_TR_REF
  Top 0.203: R11.1 72.65,29 R8.2
  Top 0.254: IC6.14 73.25,22.85 73.6,23.2 73.6,24.9 | 73.6,24.9 R15.2 | R11.1 73.4,26.73 C17.1 73.6,26.48 73.6,24.9
COMP2_OUT_DISCHARGE  (via drill 0.35)
  Top 0.203: R23.2 72.75,8.9 72.15,9.5 71.66,9.5 IC8.1
  Top 0.254: IC6.44 71.75,12.25 72.06,11.94 v72.06,11.91 | R23.2 72.9,8.9 v72,8
  Bottom 0.254: v72.06,11.91 72,11.85 v72,8
DAC1_OUT1_I_CTR_TP
  Top 0.254: IC6.15 TP1.TP
GND  (via drill 0.35, 0.6)
  Top 0.203: IC9.3 63.67,8.93 v63.7,8.9 | R26.1 72.25,3.25 73,4 75,4 v75.1,3.9 | K2.2 118,18.75 v118,17.1 116.66,15.76 116.66,8.82 117.66,7.83 117.66,4.34 118.52,3.48 X6.3 | v62.5,15 61.15,15 T2.E
  Top 0.254: IC5.2 87.22,19.12 C29.2 | C26.2 91.5,20.95 91.5,23 | IC4.2 91.5,23 | IC6.7 75.98,17.75 76.58,18.35 76.58,18.91 77.47,19.8 80.53,19.8 80.62,19.7 | 91.5,23 89.17,23 C22.2 | IC7.2 106.67,22.02 106.4,22.3 99.4,22.3 99.06,21.95 99.06,20.7 IC7.8 | 125.14,21.78 C23.2 125.12,20.12 124.88,19.88 124.5,19.88 K1.2 | IC8.2 72.19,10.25 72.56,9.88 74.73,9.88 74.95,10.1 | 66.7,3.9 v66.7,1.4 66.66,1.36 X5.9 | 66.7,3.9 66.7,4.9 66.43,5.17 X5.3 | X5.5 66.7,3.9
  Top 0.305: C27.2 99.03,20.73 99.06,20.7 | C23.2 IC3.4 IC3.5 125.12,29.15 C14.2 | LED2.C LED1.C
  Top 0.61: C32.1 C31.1 80.6,15.6 C30.2 C28.2 80.62,18.98 80.62,19.7 C25.2 80.75,20.88 v80.75,21.9 | v67.15,23.75 C16.2 C21.2 | v76.25,27.5 76.15,27.5 | C24.2 85.8,21.5 v86.1,21.8 86.2,21.9 C22.2 | v89,18.3 89,18.6 88.3,19.3 87.8,19.3 C29.2 | C19.2 IC2.2 | v132,22.5 131.3,21.8 C23.2 | C20.2 63.83,26.68 R12.2 63.85,28 v63.95,28.1 | C18.2 77.88,27.5 | 77.88,27.5 R10.1 | v76.25,27.5 77.88,27.5 | C26.2 92.97,20.45 v93.38,20.85 93.5,20.73 C27.2 | R23.1 74.95,9.9 | 74.95,9.9 74.95,10.1 74.95,10.82 C34.2 | v76.15,9.9 74.95,9.9 | R22.2 v64.75,14.12 | R11.2 76.25,28.25 v76.25,27.5 | C17.2 76.25,26.7 v76.25,27.5
  Bottom 0.203: v64.75,14.12 63.38,14.12 v62.5,15
  Bottom 0.254: v86.1,21.8 86,21.9 v80.75,21.9
  other vias: 132,31.5 132,26.5 132,18.5 170,51.38 170,50.08 170,48.77 170,47.48 170,46.17 170,44.88 170,43.58 170,42.27 170,40.98 170,39.67 170,38.38 170,37.08 170,35.77 170,34.48 170,1.5 170,2.8 170,4.1 170,5.4 170,6.7 170,8 170,9.3 170,10.6 170,11.9 170,13.2 170,14.5 170,15.8 170,17.1 170,18.4 188,37.38 186,35.38 184,37.38 182,35.38 178,35.38 176,37.38 174,35.38 172,37.38 168,37.38 166,35.38 164,37.38 162,35.38 160,37.38 158,35.38 156,37.38 154,35.38 152,37.38 150,35.38 148,37.38 146,35.38 168,15.5 166,17.5 164,15.5 162,17.5 160,15.5 158,17.5 156,15.5 154,17.5 152,15.5 150,17.5 148,15.5 146,17.5 144,15.5 172,15.5 174,17.5 176,15.5 178,17.5 182,17.5 184,15.5 186,17.5 188,15.5 142,17.5 140,15.5 138,17.5 136,15.5 142,35.38 140,37.38 138,35.38 136,37.38 134,35.38 93.4,18.3 180,51.38 180,50.08 180,48.77 180,47.48 180,46.17 180,44.88 180,43.58 180,42.27 180,40.98 180,39.67 180,38.38 180,37.08 180,35.77 180,34.48 180,1.5 180,2.8 180,4.1 180,5.4 180,6.7 180,8 180,9.3 180,10.6 180,11.9 180,13.2 180,14.5 180,15.8 180,17.1 180,18.4 115,29 117.5,29 119.2,26.3 116.1,26.3 108.2,23.7 113,30 113,27.8 108.2,28.4 108.2,31 98.4,30 95.45,30 92.35,30 89.3,30 91.25,31.5 85,30.25 90.8,30 93.9,30 97,30 98.15,27.6 98.25,25.65 103.95,26.85 108.2,25.9 101.75,24.15 120,29
  pour Bottom: 63.45,0 63.45,36.4 127.5,36.4 127.5,41.5 123.75,41.5 122.5,42.75 122.5,51.5 124,53 127.5,53 190,53 190,0 127.5,0 127.5,10.8 83.1,10.8 79.5,7.2 79.5,0
  pour Top (isolate 0.305): 190,53 127.5,53 127.5,0 190,0
  pour Top (isolate 0.406, no thermals): 80.67,30.9 80.67,32.8 81.08,33.2 98.3,33.2 98.6,32.9 98.6,30.7 99.3,30 105.55,30 105.9,30.35 105.9,31.2 105.95,31.15 115.05,31.15 115.45,31.55 115.45,32.5 115.5,32.45 119.55,32.45 120.5,31.5 121,31.5 122.45,30.05 122.45,25.95 122,25.5 121.95,25.5 119.5,23.05 97.56,23.05 96.4,24.21 96.4,27.1 95,28.5 80.7,28.5
  pour Route2: 79.5,0 63.45,0 63.45,36.4 127.5,36.4 127.5,53 190,53 190,0 127.5,0 127.5,10.8 83.1,10.8 79.5,7.2
  pour Route3: 79.5,0 63.45,0 63.45,36.4 127.5,36.4 127.5,53.05 190,53.05 190,0 127.5,0 127.5,10.8 83.1,10.8 79.5,7.2
GND2  (via drill 0.35)
  Top 0.203: IC7.9 99.06,7.3 X4.5 | v106.75,6.5 106.75,11.32 IC7.15
  Top 0.254: IC7.15 106.67,13.28 | 106.67,13.28 106.67,14 108.17,15.5 C33.1 111.22,15.9 113.91,15.9 D6.A | IC7.9 99.06,12.76 99.58,13.28 106.67,13.28
  Bottom 0.203: X3.5 97.8,3.48 X4.5 | X6.5 120.02,4.75 108.5,4.75 v106.75,6.5
IS-
  Top 0.203: IC1.4 104.05,34.25 104.7,34.9 R4.1 106.55,34.15 C10.1 109.42,35.12 R5.2
  pour Top (no thermals): 103.75,42.5 111.88,42.5 111.88,33.38 103.75,33.38
LED_ERROR  (via drill 0.35)
  Top 0.203: R17.1 111.5,19.2 v110.8,18.5
  Top 0.254: v71.6,18.7 71.8,18.5 71.8,16.4 70.25,14.85 IC6.41
  Bottom 0.203: v71.6,18.7 75.4,18.7 77.3,16.8 82.1,16.8 82.87,17.57 109.87,17.57 v110.8,18.5
LED_FUNC  (via drill 0.35)
  Top 0.203: R18.1 114.5,21 v112,18.5
  Top 0.254: v71.05,17.8 71.05,16.4 69.75,15.1 IC6.40
  Bottom 0.203: v71.05,17.8 75.65,17.8 77.06,16.39 82.37,16.39 83.14,17.16 110.66,17.16 v112,18.5
LPUART1_DE  (via drill 0.35)
  Top 0.254: IC7.5 103.5,20.6 | 103.5,20.6 IC7.4 | v103.5,18.88 103.5,20.6 | v69.7,19.65 68.85,19.65 67.3,21.2 65.6,21.2 64.25,19.75 64.25,17.5 66,15.75 IC6.34
  Bottom 0.254: v103.5,18.88 102.78,19.6 78.97,19.6 78.58,20 70.05,20 v69.7,19.65
LPUART1_RX  (via drill 0.35)
  Top 0.254: v105.35,18.85 105.41,18.91 IC7.3 | IC6.32 67.55,16.75 v68.25,17.45
  Bottom 0.254: v105.35,18.85 104.1,20.1 79.3,20.1 78.93,20.47 68.97,20.47 68.25,19.75 v68.25,17.45
LPUART1_TX  (via drill 0.35)
  Top 0.254: IC7.6 v101.6,18.85 | IC6.29 68.5,18.25 v69,18.75
  Bottom 0.254: v101.6,18.85 101.4,19.05 78.71,19.05 78.26,19.5 70.65,19.5 69.9,18.75 v69,18.75
LVP  (via drill 0.35)
  Top 0.203: R19.1 117.3,21.25 115.75,21.25 113.2,18.7 v113.2,18.5
  Top 0.254: IC6.38 68.75,15.45 69.05,15.75 69.05,16.82 69.8,17.57 v69.8,17.77
  Bottom 0.203: v69.8,17.77 70.6,16.98 75.8,16.98 76.79,15.99 82.64,15.99 83.4,16.75 111.45,16.75 v113.2,18.5
LVP_IN  (via drill 0.35)
  Top 0.254: K1.4 126.38,11.49 v126.38,1.38
  Bottom 0.203: X3.1 84.59,3.41 87.03,0.97 125.84,0.97 126.25,1.38 v126.38,1.38
LVP_OUT  (via drill 0.35)
  Top 0.203: K1.3 123.86,11.85 125.62,10.08 v125.62,3.12
  Bottom 0.203: X4.1 109.25,2.19 122.76,2.19 123.7,3.12 v125.62,3.12
N$1
  Top 0.203: IC3.6 124.47,28.35 124.33,28.5 124.33,29.79 123.5,30.62 R6.1
N$2
  Top 1.016: R2.1 R1.2
  pour Top (no thermals): 100.95,47.75 103.9,47.75 104,47.65 104,43.55 103.65,43.2 100.85,43.2 100.85,47.65
N$3
  Top 0.254: IC6.8 74.2,18.25 73.86,17.91 73.86,16.28 74,16.14 74,14.5 74.25,14.25 77.55,14.25 C31.2 78.8,12.38 Q1.2
N$4
  Top 0.203: L1.2 85.25,28.25 86.8,28.25
  Top 0.305: IC2.1 86.8,28.25 D5.A
N$5
  Top 1.016: 99.48,48.98 C1.2
  Top 1.778: R1.1 99.48,48.98
N$6
  Top 0.254: IC4.4 89.25,23.95 88.9,23.6 C22.1
N$7  (via drill 0.6)
  Top 1.422: C4.- 87.95,50.55 v86.55,50.55 | v107.35,47.75 107.35,47.05 | 107.35,47.05 v107.35,46.4 | T1.4 107.33,47.03 107.35,47.05
  Bottom 1.422: v107.35,46.4 v107.35,47.75 102.45,47.75 99.65,50.55 v86.55,50.55 v86.55,49.1
  pour Top (no thermals): 90.25,51.66 90.25,47.25 89.25,46.25 85.25,46.25 85,46.5 85,49.5 84.5,50 79.75,50 79.75,40.75 75.25,40.75 75.25,50 71.25,50 71.25,46.75 68.5,46.75 68.5,51.74
N$8  (via drill 0.35)
  Top 0.254: IC8.4 v66.5,10.9 | v77.08,24.11 77.08,22.66 v76.2,21.79 | v124.35,20.7 124.23,20.82 124.23,22.5 123.83,22.9 IC3.2
  Bottom 0.254: v66.5,10.9 66.35,11.05 66.35,14.65 65.75,15.25 65.73,20.53 69.56,24.36 75.75,24.38 76.02,24.11 v77.08,24.11 | v76.2,21.79 76.21,21.8 79.21,21.8 80.05,22.63 122.42,22.63 v124.35,20.7
N$9  (via drill 0.35)
  Top 0.254: IC6.9 73.8,18.75 73.35,18.3 73.35,14.6 v73.25,14.5 | R21.2 v89.5,15.5
  Bottom 0.254: v89.5,15.5 89.1,15.1 73.85,15.1 v73.25,14.5
N$10
  Top 0.203: 55.75,7 SP1.P$2 56.25,7 56.25,13.88 56.38,14 T2.C
N$11
  Top 1.422: T1.7 110.97,47.03 108.49,49.51 T1.5
N$12
  Top 0.254: R21.1 86.5,15.5 | 86.5,15.5 C32.2 | Q1.1 88.08,13.92 86.5,15.5
N$14  (via drill 0.35)
  Top 0.203: v105.3,30.07 105.32,30.05 IC1.1
  Top 0.254: R13.2 R14.2
  Top 0.61: R13.2 71.97,27.88 v72,27.88
  Route3 0.203: v105.3,30.07 105.3,29.6 100.47,24.77 | 100.47,24.77 99.3,23.6 v99.3,23.4 | 100.47,24.77
  Bottom 0.254: v72,27.88 74.04,25.86 81.86,25.86 83.5,24.21 83.49,24.21 84.5,23.2 99.1,23.2 v99.3,23.4
N$16
  Top 0.254: R28.2 59.15,12.4 59.8,13.05 T2.B
N$17
  Top 1.016: R2.2 97.62,44.7 D1.C
  pour Top (no thermals): 100.25,44.95 100.25,41.75 97.25,38.75 76.5,38.75 76,39.25 73.75,39.25 73.27,39.73 68.5,39.73 68.5,45.51 71.68,45.51 71.68,49.25 74.75,49.25 74.75,40.25 80.5,40.25 80.5,49.5 84,49.5 84.25,49.25 84.25,46.25 85,45.5 89.47,45.5 91.26,47.25 97.95,47.25
N$18
  Top 0.254: R20.2 LED4.A
N$19
  Top 0.254: LED3.A 117.75,23.4 R19.2
N$20
  Top 0.254: R6.2 122.65,31.6 120.28,31.6 T3.G
N$21
  Top 0.254: JP1.3 75.36,2.39 74.75,3 R26.2
N$22
  Top 0.254: IC5.1 85.78,18.07 87.28,18.07 C29.1
N$23
  Top 1.016: C11.1 121.85,32.52 121.85,33.78 122.25,34.18 R3.1
N$24  (via drill 0.35)
  Top 0.254: R9.2 77.88,30.38 v77.88,31.62 | v123.88,37.5 123.88,39.12 120.4,39.11 120.88,39.59
  Bottom 0.254: v77.88,31.62 77.88,35.5 80,37.5 v123.88,37.5
  pour Top (no thermals): 122.25,43.5 112.5,43.5 112.5,33.62 120.5,33.62 120.5,35.75 122.25,35.75
N$25
  Top 1.016: C10.2 110.33,32.45 R5.1 113.52,32.28 D4.C
N$26  (via drill 0.35)
  Top 0.203: R28.1 62.82,11.5 63.19,11.88 63.19,14.69 63.21,14.71 63.21,15.83 v63.62,16.25 | v65.01,17.78 66.72,17.78 IC6.30
  Bottom 0.203: v65.01,17.78 63.62,16.4 v63.62,16.25
N$28
  pour Top: 57.5,52.12 67.5,52.12 67.5,41.62 67.62,41.5 57.5,41.5
N$31
  Top 0.254: R18.2 LED2.A
N$34
  Top 0.254: R17.2 LED1.A
N$35
  Top 0.203: LED4.C 121.68,25.07 121.68,19.5 121.03,18.85 K2.1
N$36
  Top 0.203: LED3.C 117.75,26.5 118.52,27.29 121.97,27.29 122.25,27.01 122.25,17.75 122.5,17.5 124.67,17.5 K1.1
NRST  (via drill 0.35)
  Top 0.254: C25.1 77.6,20.75 76.1,19.25 IC6.10 73.45,19.25 72.85,18.65 72.85,15.38 72.12,14.65 v72.12,14.5 | R27.1 71.03,1.43 v71,1.4 68.79,1.4 X5.10
  Bottom 0.254: v71,1.4 71.1,1.4 73.03,3.32 73.03,12.5 72.12,13.4 v72.12,14.5
OVP  (via drill 0.35)
  Top 0.203: R20.1 120.45,21.65 119.4,20.6 115.75,20.6 114.25,19.1 v114.25,18.5
  Top 0.254: v69.95,16.52 69.95,15.95 69.25,15.25 IC6.39
  Bottom 0.203: v69.95,16.52 75.55,16.52 76.49,15.58 82.91,15.58 83.67,16.35 112.1,16.35 v114.25,18.5
OVP_IN  (via drill 0.35)
  Top 0.203: K2.4 121.27,11.85 122.39,10.72 124.14,10.72 124.88,10 v124.88,2.12
  Bottom 0.203: X3.3 87.12,2.73 88.48,1.38 124.12,1.38 v124.88,2.12
OVP_OUT  (via drill 0.35)
  Top 0.203: v123.75,2.12 124.25,2.62 124.25,9.83 123.86,10.23 120.11,10.23 118.48,11.85 K2.3
  Bottom 0.203: X4.3 104,4.89 104,2.62 104.84,1.78 123.41,1.78 v123.75,2.12
R1  (via drill 0.35)
  Top 0.203: v70.4,11.8 70.75,12.15 IC6.42 | v71,3.74 70.84,3.9 X5.6
  Bottom 0.203: v71,3.74 70.24,4.5 70.24,11.64 v70.4,11.8
R2  (via drill 0.35)
  Top 0.203: IC6.37 67.2,13.25 v67.15,13.3
  Top 0.254: X5.8 70.97,2.63 v71,2.6
  Bottom 0.254: v67.15,13.3 67.15,12 67.4,11.75 67.4,6.2 v71,2.6
SWCLK
  Top 0.203: X5.4 67.33,5.17 66.75,5.75 66.75,7 64.75,9 R22.1 arc60 64.75,11.25 65.75,11.25 65.88,11.38 65.88,14.62 66,14.75 IC6.36
SWDIO  (via drill 0.35)
  Top 0.254: X5.2 v65.62,9.62 | IC6.35 65.75,15.25 65.62,15.38 v65,15.38
  Bottom 0.203: v65.62,9.62 65.62,14.38 65,15 v65,15.38
VCC  (via drill 0.35)
  Top 0.203: C34.1 73.17,10.9 IC8.3 71.42,10.75 70.84,10.75 70.34,10.25 IC8.5
  Top 0.254: C24.1 83.08,21.5 | C28.1 77.83,18.95 v77.62,18.75 76.12,17.25 IC6.6 74.54,17.25 74.32,17.03 74.32,16.47 74.51,16.27 75.22,16.27 IC6.4 | IC7.7 100.33,18.9 | 100.33,18.9 100.33,18.68 101,18 106.7,18 107.94,19.25 IC7.1 | C27.1 96.97,18.9 100.33,18.9 | IC1.5 104.15,30.05 104.42,29.77 C15.1 | C34.1 73.22,11.05 74.47,12.3 v74.95,12.3 | IC9.1 64.17,7.98 v64.35,7.8 64.35,6.94 X5.1 | v75.25,1.25 75.08,1.43 R27.2
  Top 0.305: C26.1 90.3,19.85 90.9,19.25 96.62,19.25 C27.1 | v82.95,23.45 84.35,23.45 v84.9,24 | C15.1 v103.22,28.6
  Top 0.61: 83.08,21.5 IC5.4 84.38,20.07 | 84.38,20.07 IC5.3 85.86,20.07 86.44,20.65 89,20.65 89.2,20.45 C26.1 90.3,22.05 IC4.5 | v82.95,23.45 83.12,23.27 C24.1 | 84.38,20.07 v84.38,18.27
  Route3 0.305: v98.3,24 98.65,24 103.22,28.57 v103.22,28.6
  Route3 0.406: v75.25,1.25 74,2.5 74,11.35 v74.95,12.3 74.35,12.9 69.85,12.9 v68.75,11.8
  Route3 0.61: v64.35,7.8 66.3,7.8 68.75,10.25 v68.75,11.8
  Bottom 0.254: v84.38,18.27 84.28,18.38 78,18.38 v77.62,18.75
  Bottom 0.305: v84.9,24 v98.3,24
  Bottom 0.61: v82.95,23.45 83,23.4 79.65,23.4 78.95,22.7 70,22.7 67,19.7 67,15.65 68.75,13.9 v68.75,11.8
VCC2  (via drill 0.35)
  Top 0.203: IC7.16 107.94,2.45 107.5,2 101.81,2 X4.6 | D6.C 114.5,12.32 v114.5,9.5
  Top 0.254: IC7.16 107.94,12.82 108.35,13.22 110.3,13.22 110.7,12.82 | 110.7,12.82 C33.2 | D6.C 114.45,12.82 110.7,12.82
  Bottom 0.203: X3.6 98.39,6.02 99.5,7.12 101,7.12 101.5,6.62 101.5,4.64 X4.6 | X6.6 121.29,8.21 120,9.5 v114.5,9.5
VIN
  Top 0.203: R4.2 101.5,34.9 102.2,34.2 102.2,31.7 102.8,31.1 104.8,31.1 105.65,31.95 IC1.3 | 69.47,31.12 69.4,31.05 R8.1 R7.2
  Top 0.254: F1.2B 75.98,31.12 69.47,31.12
  Top 0.61: L1.1 81.65,27 C13.1 81.65,36.01 81.62,36.03 | F1.2B 76.2,36.03 | F1.2A 76.2,37.41 76.2,36.03 | 81.62,36.03 D3.C 87.75,36.03 C6.1 C8.1 C9.1 | 81.62,36.03 76.2,36.03
  pour Top (isolate 0.406, no thermals): 99.4,31.2 101,31.2 101.2,31.4 101.2,36.3 101,36.5 83.4,36.5 82.4,37.5 76.6,37.5 76.4,37.7 72.4,37.7 72.4,34.3 72.7,34 98.3,34 99.3,33 99.3,31.3
VREF  (via drill 0.35)
  Top 0.254: R24.1 71.35,6.6 70.25,7.7 v68.95,7.7 | v81.75,24.38 81.75,22.25 81.76,19.1 | C30.1 77.89,17.35 v77.64,17.61 76.78,16.75 IC6.5 | 81.76,19.1 81.76,18.2 | 81.76,18.2 v81.76,17.55 | IC5.6 81.78,18.18 81.76,18.2 | IC5.5 81.78,19.12 81.76,19.1 | R15.1 75.25,25.1 v75.25,23.62
  Bottom 0.254: v81.75,24.38 81.5,24.12 79.38,24.12 78.62,23.38 75.5,23.38 75.2,23.65 | 75.2,23.65 75.25,23.65 v75.25,23.62 | 75.2,23.65 69.72,23.65 66.28,20.21 66.28,15.38 68,13.66 68,8.65 v68.95,7.7 | v77.64,17.61 77.69,17.55 v81.76,17.55
VREF_
  Top 0.254: JP1.1 75.92,7.46 75.06,6.6 R24.2

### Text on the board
tPlace: ECS | - | + | www.ecs-online.org | ERROR | FUNC | LVP | OVP | IN | OUT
